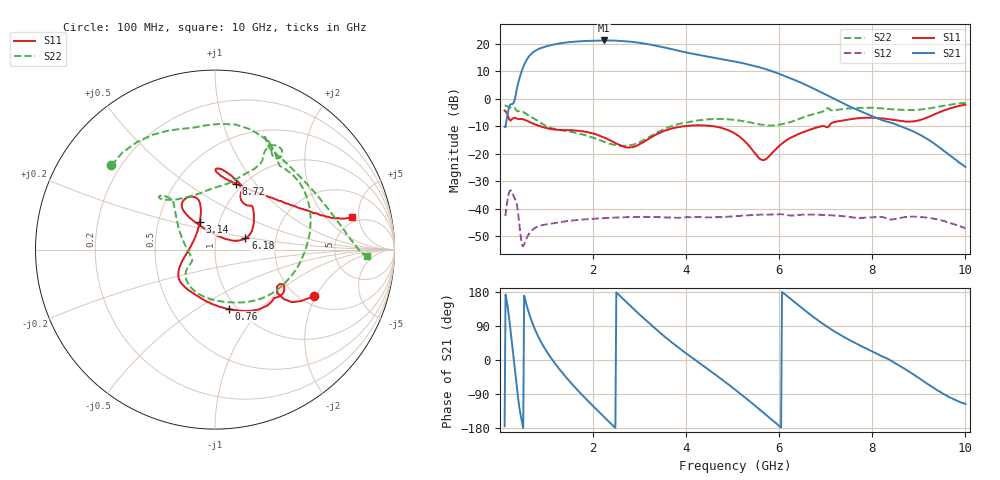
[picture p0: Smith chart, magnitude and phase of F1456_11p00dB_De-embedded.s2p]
! Integrated Device Technology
! Corporate Headquarters
! 6024 Silver Creek Valley Road
! San Jose, CA 95138  USA
! Phone:  1-408-284-8200
! Toll Free:  1-800-223-1366
! Webpage:  http://www.idt.com/
! Timing and RF Division
! 515 Groton Road, Suite 102
! Westford, MA 01886-6024
! Device:  F1456
! Description: 6-bit 0.5 dB Transmit Variable Gain Amplifier
! Frequency:  2100.0 -  2950.00 MHz
! Package:  6x6 mm Thin QFN Plastic Package: 28 pin
! State:  22
! Atten State:  11.0 dB
! Voltage:  +5.00 Volts
! Current:  217.020 mA
! Data:  The device was measured on a the F1455 evaluation board which has
!  individual transmission lines to the RF pins.  Data was collected
!  using a calibrated network analyzer.  The evaluation board was
!  de-embedded using a TRL calibration technique.
!  The reference plane is the edge of the package pin.
!  Pin  1 = CSb
!  Pin  2 = DATA
!  Pin  3 = CLK
!  Pin  4 = RSET
!  Pin  5 = GND
!  Pin  6 = RFIN  = Port 1
!  Pin  7 = GND
!  Pin  8 = NC
!  Pin  9 = NC
!  Pin 10 = NC
!  Pin 11 = NC
!  Pin 12 = NC
!  Pin 13 = NC
!  Pin 14 = /STBY
!  Pin 15 = GND
!  Pin 16 = RFOUT  = Port 2
!  Pin 17 = GND
!  Pin 18 = NC
!  Pin 19 = NC
!  Pin 20 = NC
!  Pin 21 = GND
!  Pin 22 = NC
!  Pin 23 = GND
!  Pin 24 = NC
!  Pin 25 = NC
!  Pin 26 = NC
!  Pin 27 = GND
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# GHz S dB R 50
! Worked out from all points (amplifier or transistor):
!   496 points, 100 MHz to 10 GHz, reference 50 ohm
!   highest |S21| = 21.2 dB at 2.24 GHz (marker M1)
!   |S21| within 3 dB of that: 846.9 MHz to 3.649 GHz (2.802 GHz wide, 125 % of centre)
!   unconditionally stable (mu >= 1): start of sweep to end of sweep
!   at 1.74 GHz: K = 6.42, MAG = 21.5 dB, |S12| = -44.1 dB
!   at 5.06 GHz: K = 11.54, MAG = 14.5 dB, |S12| = -42.8 dB
!   at 10 GHz: K = 218.79, MAG = -15.2 dB, |S12| = -47.1 dB
!   S11 on the Smith chart (normalised r, x): 100 MHz: 2.34, -1.94; 760 MHz: 0.92, -0.68; 3.14 GHz: 0.81, +0.25; 6.18 GHz: 1.39, +0.18; 8.72 GHz: 0.94, +0.80; 10 GHz: 4.29, +4.03
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0.1  -4.28 -25.2  -10.18 -175.0  -42.30 46.6  -2.57 140.9
0.32  -6.92 -32.4  -0.17 -20.7  -36.44 -140.8  -3.38 65.4
0.44  -7.36 -42.9  8.61 -142.4  -49.31 139.9  -4.41 38.9
0.58  -8.02 -59.0  14.36 141.6  -50.58 173.3  -5.69 4.9
0.76  -9.41 -77.1  17.50 78.6  -47.04 131.9  -7.53 -30.1
0.98  -10.60 -97.8  19.01 27.1  -45.82 91.1  -9.83 -66.1
1.2  -11.28 -114.4  19.93 -11.8  -45.25 65.8  -11.09 -93.2
1.5  -11.47 -131.5  20.65 -56.9  -44.47 40.0  -11.99 -121.0
1.76  -11.82 -142.1  20.98 -91.5  -44.03 22.1  -12.93 -136.1
2.24  -14.13 -159.9  21.25 -150.5  -43.51 -5.6  -15.68 -149.2
2.64  -17.39 170.6  21.04 161.8  -43.21 -26.8  -17.19 -159.3
3.14  -15.14 119.2  20.02 104.2  -43.05 -52.2  -14.56 163.3
3.4  -12.67 109.8  19.18 76.1  -43.15 -64.7  -12.11 146.1
3.72  -10.73 108.3  17.97 43.7  -43.34 -78.9  -9.76 134.0
4.08  -9.79 114.2  16.59 10.4  -43.22 -93.6  -8.44 131.1
5.06  -12.79 128.6  13.51 -78.9  -42.80 -135.4  -7.73 136.6
5.64  -22.29 71.2  11.16 -136.9  -42.25 -166.8  -9.52 120.0
6.18  -14.87 20.3  7.83 167.8  -42.41 160.0  -8.75 82.0
6.7  -11.04 39.2  4.03 116.8  -42.22 132.1  -5.78 63.4
8.36  -7.45 87.6  -8.54 1.2  -43.89 60.6  -3.79 62.5
8.72  -8.32 72.1  -10.70 -25.5  -43.10 52.1  -4.08 50.4
10  -2.13 13.5  -24.78 -116.2  -47.13 -27.7  -1.46 -2.5
